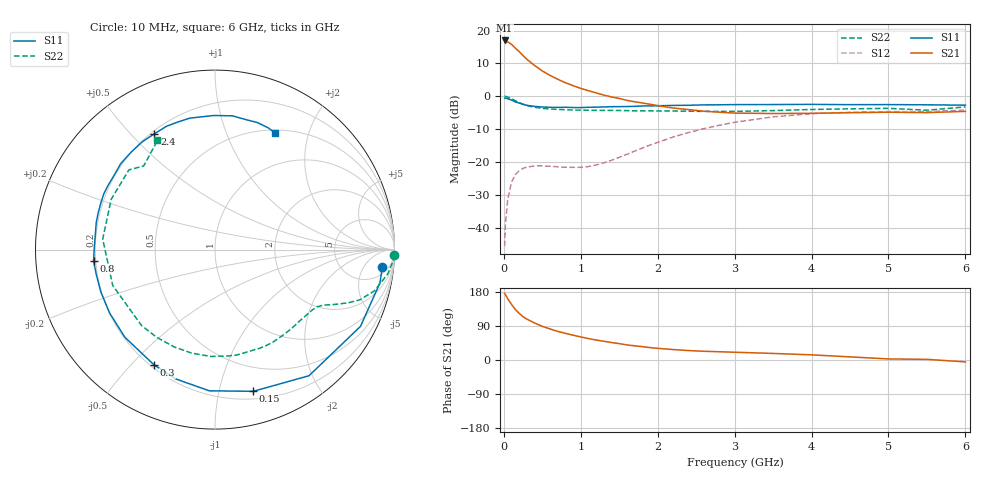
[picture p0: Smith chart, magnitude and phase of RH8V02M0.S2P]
! SIEMENS Small Signal Semiconductors
! BFR106
! Si NPN RF Bipolar Junction Transistor in SOT23
! VCE = 8 V  IC = 2 mA
! Common Emitter S-Parameters:  August  1996
# GHz  S  MA  R  50
!  f  S11  S21  S12  S22
! GHz  MAG  ANG  MAG  ANG  MAG  ANG  MAG  ANG
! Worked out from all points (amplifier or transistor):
!   36 points, 10 MHz to 6 GHz, reference 50 ohm
!   highest |S21| = 17.0 dB at 10 MHz (marker M1)
!   |S21| within 3 dB of that: start of sweep to 180.6 MHz
!   unconditionally stable (mu >= 1): 796.1 MHz to 1.807 GHz; 4.144 GHz to end of sweep
!   at 250 MHz: K = 0.32, MSG = 17.2 dB, |S12| = -22.0 dB
!   at 1.4 GHz: K = 1.23, MAG = 6.7 dB, |S12| = -19.5 dB
!   at 6 GHz: K = 1.02, MAG = -1.1 dB, |S12| = -4.2 dB
!   S11 on the Smith chart (normalised r, x): 10 MHz: 9, -14; 150 MHz: 0.27, -1.27; 300 MHz: 0.21, -0.58; 800 MHz: 0.19, -0.04; 2.4 GHz: 0.21, +0.59; 6 GHz: 0.53, +1.50
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0.01  0.9375 -5.8  7.075 175.6  0.0052 87.9  0.9992 -1.7
0.02  0.9375 -11.4  6.992 172.9  0.011 81.3  0.996 -3.3
0.05  0.9166 -27.8  6.746 161.7  0.0267 74.8  0.9723 -8.0
0.1  0.8765 -53.3  6.168 146.8  0.0489 62.3  0.9177 -14.5
0.15  0.8178 -74.9  5.402 132.9  0.0642 51.4  0.8545 -19.1
0.2  0.7874 -92.3  4.774 123.1  0.0736 44.2  0.8008 -21.7
0.25  0.7531 -106.8  4.163 114.2  0.0797 38.3  0.7536 -23.7
0.3  0.7265 -117.9  3.65 107.9  0.0834 34.7  0.7229 -25.1
0.4  0.7005 -135.8  2.941 97.5  0.0866 29.8  0.6786 -27.1
0.5  0.6854 -148.9  2.43 88.8  0.0866 27.9  0.6528 -29.2
0.6  0.6784 -159.6  2.078 81.9  0.0856 28.1  0.6387 -31.6
0.8  0.6794 -174.7  1.606 70.4  0.083 32.6  0.6227 -37.1
1.1  0.6785 167.2  1.213 56.5  0.0848 48.1  0.6115 -46.8
1.6  0.6964 145.4  0.864 39.8  0.1304 70.7  0.6036 -65.6
2.2  0.7246 124.0  0.661 27.6  0.2387 72.1  0.5958 -92.3
2.4  0.7283 117.6  0.626 24.9  0.2798 69.1  0.5913 -102.7
3  0.7458 100.8  0.554 20.5  0.401 56.4  0.5888 -134.0
3.5  0.7472 90.6  0.545 17.3  0.4855 44.1  0.6039 -160.7
4.5  0.7444 76.8  0.561 8.2  0.5697 21.0  0.6427 154.1
5  0.7462 71.5  0.571 2.8  0.5841 12.1  0.6538 137.2
5.5  0.7402 66.2  0.563 1.7  0.5842 7.6  0.6123 130.4
6  0.731 63.0  0.588 -5.0  0.6144 -0.7  0.6877 117.8
